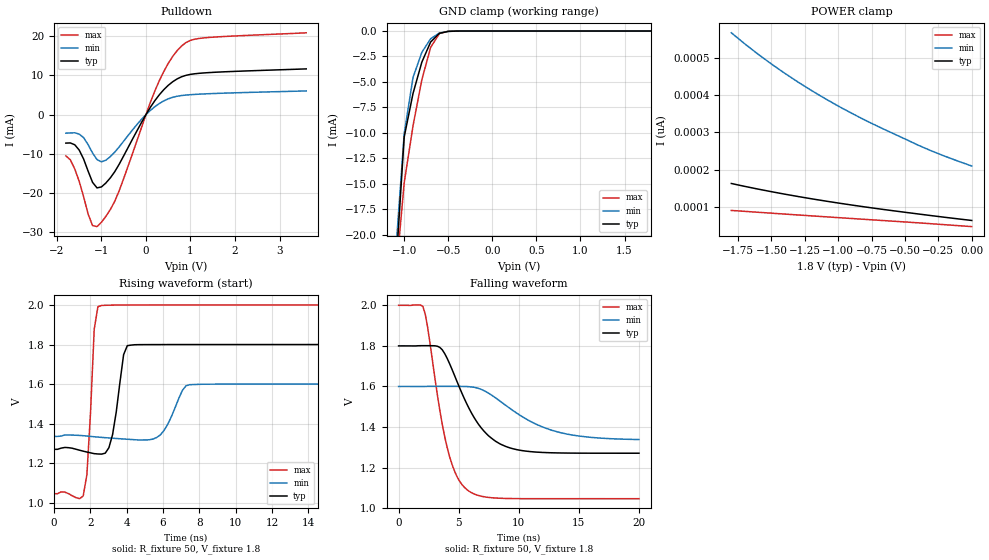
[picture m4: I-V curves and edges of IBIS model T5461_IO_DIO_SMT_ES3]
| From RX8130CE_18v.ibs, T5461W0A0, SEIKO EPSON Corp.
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[Model]   T5461_IO_DIO_SMT_ES3
Model_type I/O_open_drain
Enable Active-High
Polarity Non-Inverting
Vinh=1.60
Vinl=0.32
Vmeas=0.90
Vref=2.0
Rref=5000
C_comp   2.5p   2.0p   3.0p
[Temperature Range] 25   85   -40
[Voltage Range]   1.8   1.6   2.0
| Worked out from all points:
|   slope of the pulldown table from 0 to 0.27 V, typ, clamps not added: 58.7 ohm
|   GND clamp passes 1 mA (typ) near -0.69 V on its own axis
|   falling waveform, R_fixture 50, V_fixture 1.8: 20-80 % time 2.78ns typ, 4.45ns min, 1.71ns max; typ from 1.8 V to 1.27 V
|   rising waveform, R_fixture 50, V_fixture 1.8: 20-80 % time 472ps typ, 757ps min, 310ps max; typ from 1.27 V to 1.8 V
[Pulldown]
-1.8V     -7.266mA   -4.736mA   -10.53mA
-1.7V     -7.222mA   -4.672mA   -11.49mA
-1.5V     -9.036mA   -4.962mA   -17.01mA
-1.2V     -17.26mA   -9.79mA    -28.27mA
-1.1V     -18.67mA   -11.46mA   -28.53mA
-900mV    -17.42mA   -11.61mA   -25.92mA
-700mV    -14.52mA   -9.554mA   -22.05mA
-100mV    -2.011mA   -1.203mA   -3.294mA
300mV     5.046mA    2.816mA    8.649mA
800mV     9.634mA    4.854mA    17.49mA
1.3V      10.61mA    5.262mA    19.53mA
3.6V      11.64mA    6.027mA    20.83mA
[GND Clamp]
-1.8V     -196.4mA   -166.6mA   -242.2mA
-1.1V     -24.06mA   -22.18mA   -24.54mA
-1V       -10.41mA   -10.09mA   -14.91mA
-900mV    -6.13mA    -4.56mA    -9.309mA
-800mV    -3.058mA   -2.096mA   -4.786mA
-700mV    -1.078mA   -757.4uA   -1.604mA
-600mV    -224.6uA   -189.6uA   -244.1uA
-500mV    -33.81uA   -37.1uA    -22.82uA
-400mV    -4.624uA   -6.222uA   -2.07uA
1.8V      65pA       236.4pA    43.61pA
[POWER Clamp]
-1.8V     163.7pA    566.2pA    91.78pA
-1.6V     148.8pA    509.2pA    86.87pA
-1.4V     135.2pA    458.1pA    82.04pA
-1.2V     122.9pA    412.1pA    77.28pA
-1V       111.6pA    370.7pA    72.57pA
-800mV    101.2pA    333.2pA    67.92pA
-400mV    82.31pA    265.9pA    58.65pA
-200mV    73.4pA     236.4pA    53.64pA
0V        65pA       210.5pA    48.62pA
[Falling Waveform]
R_fixture=50
V_fixture=1.8
V_fixture_min=1.6
V_fixture_max=2.0
0s        1.8V       1.6V       2V
2.02ns    1.801V     1.6V       1.995V
3.434ns   1.792V     1.6V       1.481V
4.04ns    1.739V     1.6V       1.299V
4.848ns   1.626V     1.6V       1.157V
5.657ns   1.516V     1.599V     1.093V
7.273ns   1.369V     1.574V     1.054V
9.293ns   1.297V     1.491V     1.047V
13.33ns   1.272V     1.374V     1.047V
20ns      1.271V     1.338V     1.047V
[Rising Waveform]
R_fixture=50
V_fixture=1.8
V_fixture_min=1.6
V_fixture_max=2.0
0s        1.271V     1.336V     1.047V
1.616ns   1.262V     1.34V      1.035V
1.818ns   1.257V     1.338V     1.142V
2.222ns   1.249V     1.334V     1.878V
2.424ns   1.247V     1.333V     1.991V
3.232ns   1.345V     1.327V     1.999V
4.04ns    1.794V     1.322V     2V
5.859ns   1.8V       1.343V     2V
7.475ns   1.8V       1.597V     2V
20ns      1.8V       1.6V       2V
[Ramp]
R_load=50
dV/dt_r   3.176E-1/4.504E-10   1.584E-1/7.479E-10   5.721E-1/2.849E-10
dV/dt_f   3.176E-1/2.776E-9   1.571E-1/4.451E-9   5.721E-1/1.705E-9
|[End   T5461_IO_DIO_SMT_ES3
